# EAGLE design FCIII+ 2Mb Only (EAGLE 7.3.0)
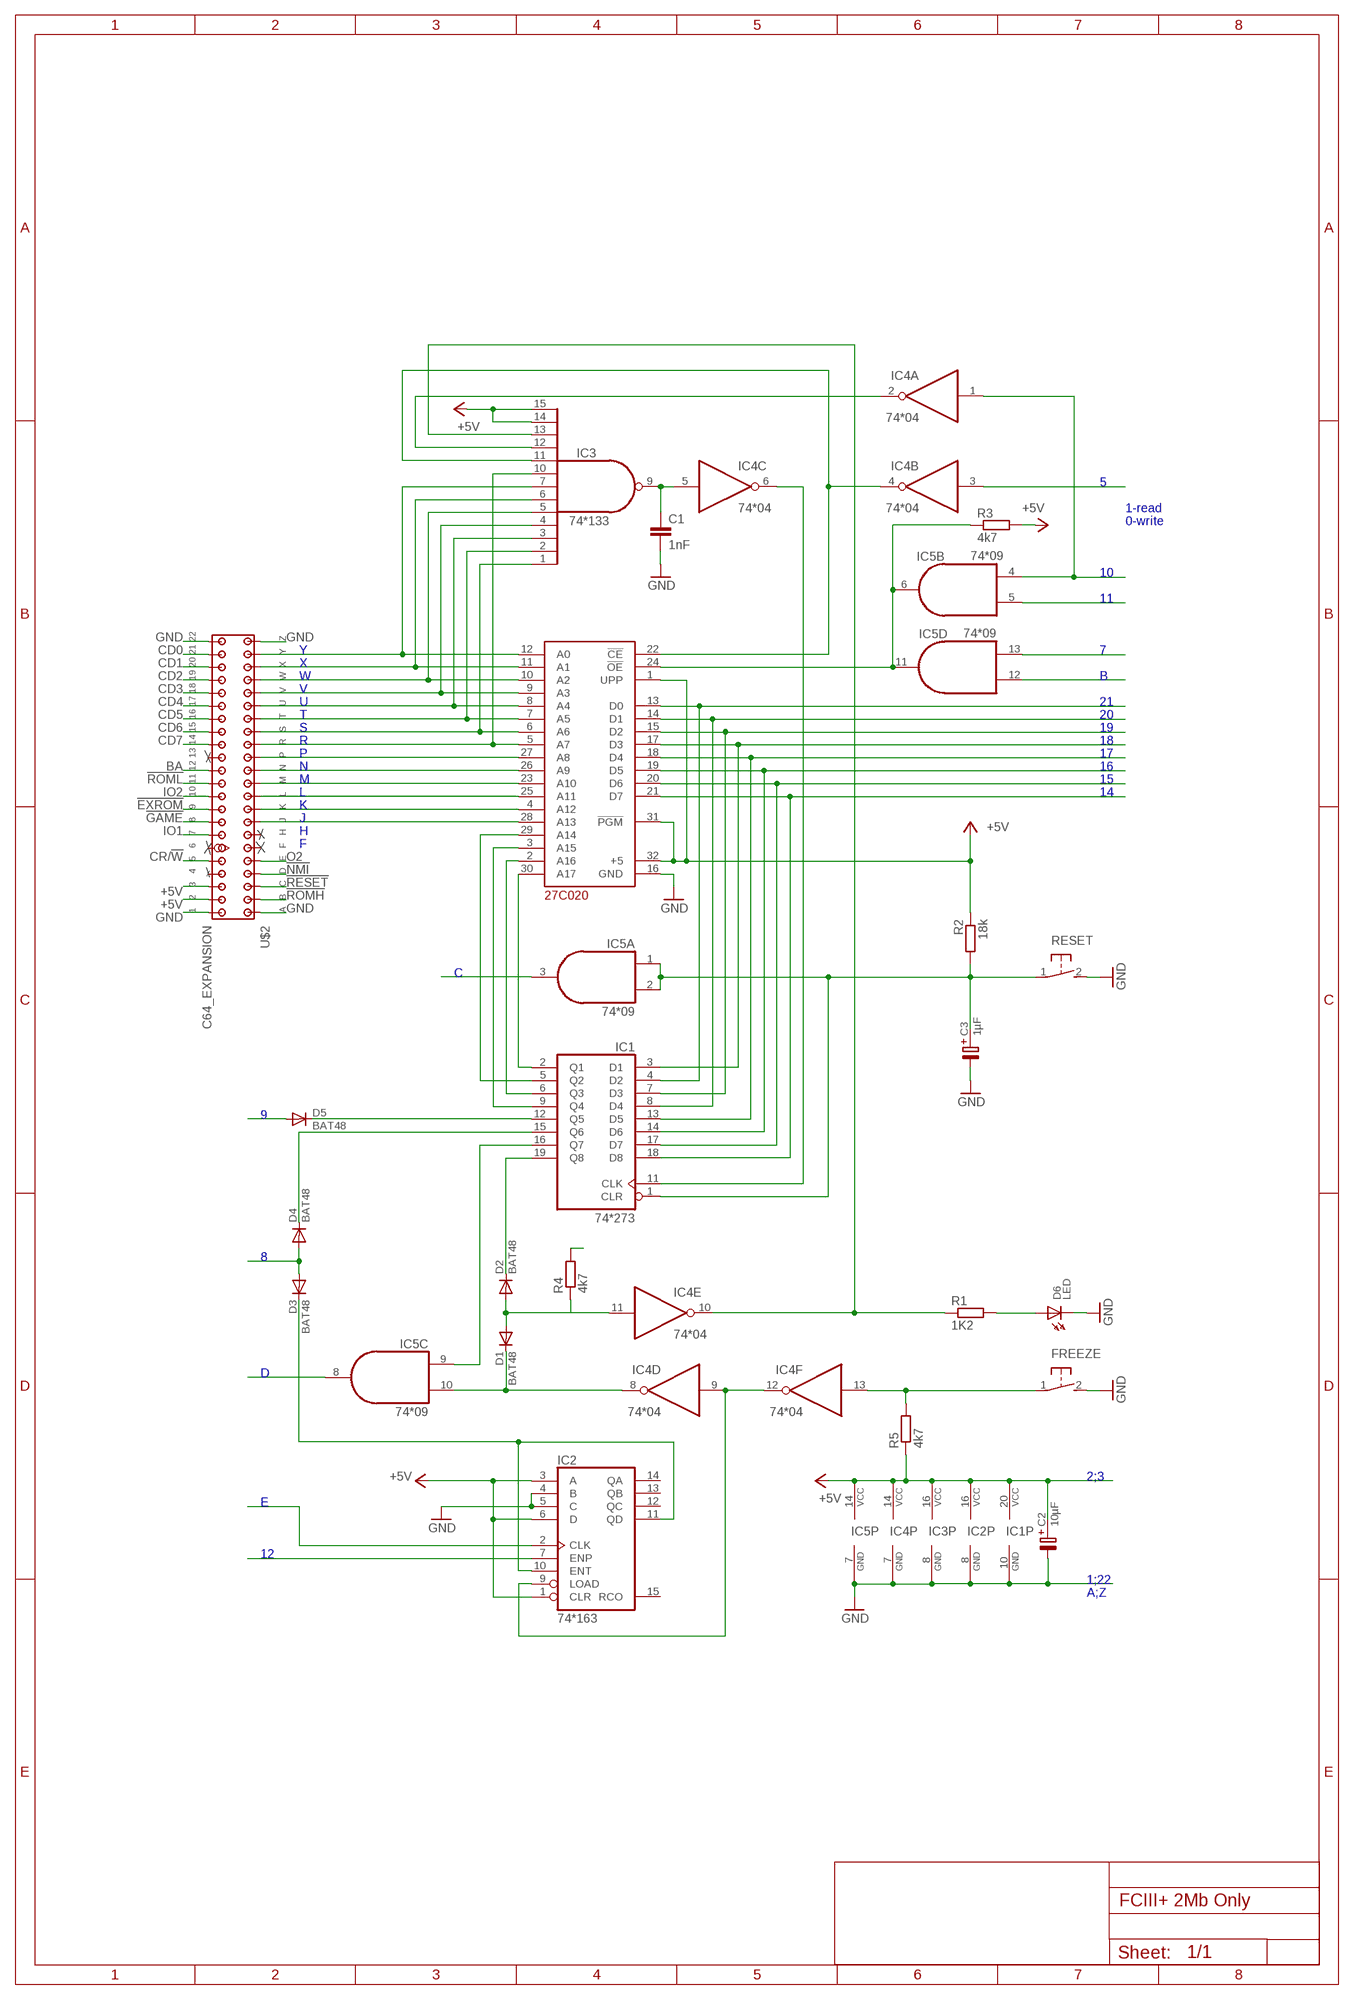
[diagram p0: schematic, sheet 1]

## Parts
C1  1nF  C-EU050-024X044  [C050-024X044]
C2  10µF  E1,6-4  [E1,6-4]
C3  1µF  E1,6-4  [E1,6-4]
D1  BAT48  OA91  [DO07]
D2  BAT48  OA91  [DO07]
D3  BAT48  OA91  [DO07]
D4  BAT48  OA91  [DO07]
D5  BAT48  OA91  [DO07]
D6  LED  LED3E  [LED3E]
FREEZE  31-XX  [B3F-31XX]
IC1  74*273  74273  [DIL20]
IC2  74*163  74160  [DIL16]
IC3  74*133  74133  [DIL16]
IC4  74*04  7404  [DIL14]
IC5  74*09  7409  [DIL14]
R1  1K2  R-EU_0207/10  [0207/10]
R2  18k  R-EU_0207/10  [0207/10]
R3  4k7  R-EU_0207/10  [0207/10]
R4  4k7  R-EU_0207/10  [0207/10]
R5  4k7  R-EU_0207/10  [0207/10]
RESET  31-XX  [B3F-31XX]
U$1  27C020  [DIL32]
U$2  C64_EXPANSION  [EDGE44_254]

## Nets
!EXROM: D5.A U$2.P$9(!EXROM)
!GAME: D3.A D4.A U$2.P$8(!GAME)
!NMI: IC5.8(C:O) U$2.D(!NMI)
!RESET: IC5.3(A:O) U$2.C(!RESET)
!ROMH: IC5.12(D:I0) U$2.B(!ROMH)
!ROML: IC5.5(B:I1) U$2.P$11(!ROML)
+5V: C2.+ IC1.20(VCC) IC2.1(CLR) IC2.3(A) IC2.6(D) IC2.16(VCC) IC3.14(I11) IC3.15(I12) IC3.16(VCC) IC4.14(P:VCC) IC5.14(P:VCC) R2.1 R3.2 R5.1 U$1.1(UPP) U$1.31(!PGM) U$1.32(+5) U$2.P$2(+5V_2) U$2.P$3(+5V_3)
BA: IC2.7(ENP) U$2.P$12(BA)
CA0: IC3.7(I6) U$1.12(A0) U$2.Y(A0)
CA1: IC3.6(I5) U$1.11(A1) U$2.X(A1)
CA2: IC3.5(I4) U$1.10(A2) U$2.W(A2)
CA3: IC3.4(I3) U$1.9(A3) U$2.V(A3)
CA4: IC3.3(I2) U$1.8(A4) U$2.U(A4)
CA5: IC3.2(I1) U$1.7(A5) U$2.T(A5)
CA6: IC3.1(I0) U$1.6(A6) U$2.S(A6)
CA7: IC3.10(I7) U$1.5(A7) U$2.R(A7)
CA8: U$1.27(A8) U$2.P(A8)
CA9: U$1.26(A9) U$2.N(A9)
CA10: U$1.23(A10) U$2.M(A10)
CA11: U$1.25(A11) U$2.L(A11)
CA12: U$1.4(A12) U$2.K(A12)
CA13: U$1.28(A13) U$2.J(A13)
CD0: IC1.4(D2) U$1.13(D0) U$2.P$21(D0)
CD1: IC1.8(D4) U$1.14(D1) U$2.P$20(D1)
CD2: IC1.7(D3) U$1.15(D2) U$2.P$19(D2)
CD3: IC1.3(D1) U$1.17(D3) U$2.P$18(D3)
CD4: IC1.13(D5) U$1.18(D4) U$2.P$17(D4)
CD5: IC1.14(D6) U$1.19(D5) U$2.P$16(D5)
CD6: IC1.17(D7) U$1.20(D6) U$2.P$15(D6)
CD7: IC1.18(D8) U$1.21(D7) U$2.P$14(D7)
CR/!W: IC4.3(B:I) U$2.P$5(R!W)
FREEZE: FREEZE.1(P) IC4.13(F:I) R5.2
GND: C1.2 C2.- C3.- D6.K FREEZE.2(S) IC1.10(GND) IC2.4(B) IC2.5(C) IC2.8(GND) IC3.8(GND) IC4.7(P:GND) IC5.7(P:GND) RESET.2(S) U$1.16(GND) U$2.A(GND_A) U$2.P$1(GND_1) U$2.P$22(GND_22) U$2.Z(GND_Z)
IO1: IC5.13(D:I1) U$2.P$7(!IO1)
IO2: IC4.1(A:I) IC5.4(B:I0) U$2.P$10(!IO2)
N$1: IC1.2(Q1) U$1.30(A17)
N$2: IC2.9(LOAD) IC4.9(D:I) IC4.12(F:O)
N$3: D1.K IC4.8(D:O) IC5.10(C:I1)
N$4: IC1.16(Q7) IC5.9(C:I0)
N$5: D3.K IC2.10(ENT) IC2.11(QD)
N$6: D5.K IC1.12(Q5)
N$7: R4.2
N$9: D1.A D2.A IC4.11(E:I) R4.1
N$10: D2.K IC1.19(Q8)
N$12: D4.K IC1.15(Q6)
N$14: IC1.6(Q3) U$1.2(A16)
N$15: IC1.9(Q4) U$1.3(A15)
N$16: IC1.5(Q2) U$1.29(A14)
N$34: C1.1 IC3.9(O) IC4.5(C:I)
N$35: IC1.11(CLK) IC4.6(C:O)
N$36: IC3.11(I8) IC4.4(B:O) U$1.22(!CE)
N$38: IC3.12(I9) IC4.2(A:O)
N$46: IC5.6(B:O) IC5.11(D:O) R3.1 U$1.24(!OE)
N$47: IC3.13(I10) IC4.10(E:O) R1.1
N$49: D6.A R1.2
O2: IC2.2(CLK) U$2.E(PHI2)
RESET: C3.+ IC1.1(CLR) IC5.1(A:I0) IC5.2(A:I1) R2.2 RESET.1(P)
Unconnected: IC2.12(QC) IC2.13(QB) IC2.14(QA) IC2.15(RCO) U$2.F(A15) U$2.H(A14) U$2.P$4(!IRQ) U$2.P$6(DOTCLK) U$2.P$13(!DMA)

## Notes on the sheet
- 5
- 1-read
- 0-write
- 10
- 11
- Y | 7
- X
- W | B
- V
- U | 21
- T | 20
- S | 19
- R | 18
- P | 17
- N | 16
- M | 15
- L | 14
- K
- J
- H
- F
- C
- 9
- 8
- D
- 2;3
- E
- 12
- 1;22
- A;Z

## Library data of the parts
C1 = rcl:C-EU: CAPACITOR, European symbol
C2 C3 = polcap:E1,6-4
D1-D5 = diode:OA91
D6 = led:LED3E
FREEZE RESET = switch-omron:31-XX: OMRON SWITCH; MPN: B3F-3100; OC_FARNELL: 959704; OC_NEWARK: 36M3582
IC1 = 74xx:74273
IC2 = 74xx:74160
IC3 = 74xx:74133
IC4 = 74xx:7404
IC5 = 74xx:7409
R1-R5 = rcl:R-EU_: RESISTOR, European symbol
U$1 = memory:27C020
U$2 = 000_e5frog:C64_EXPANSION

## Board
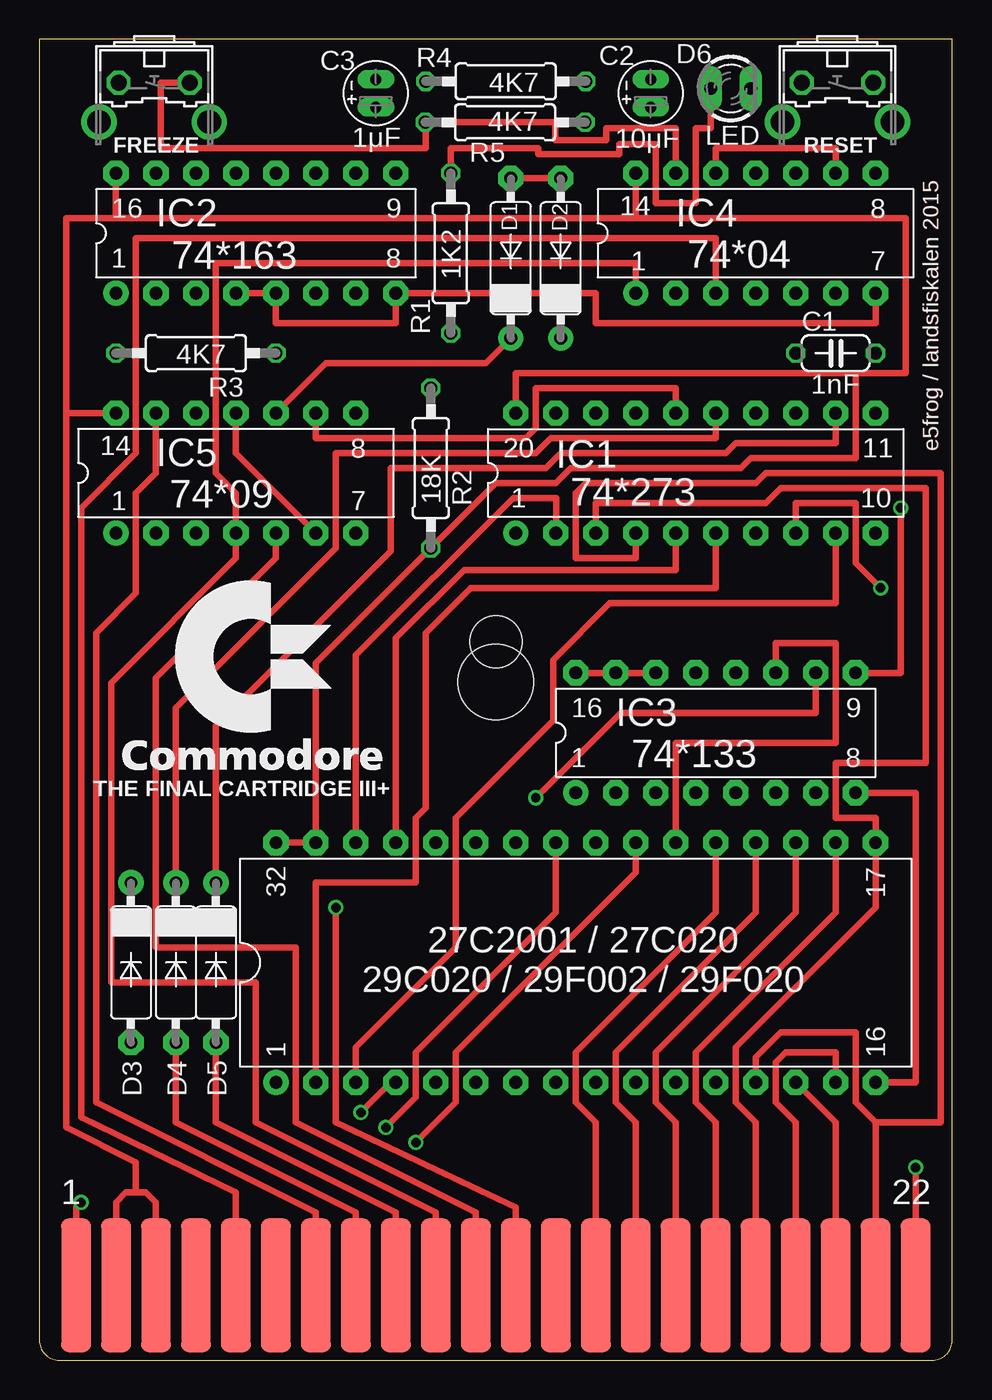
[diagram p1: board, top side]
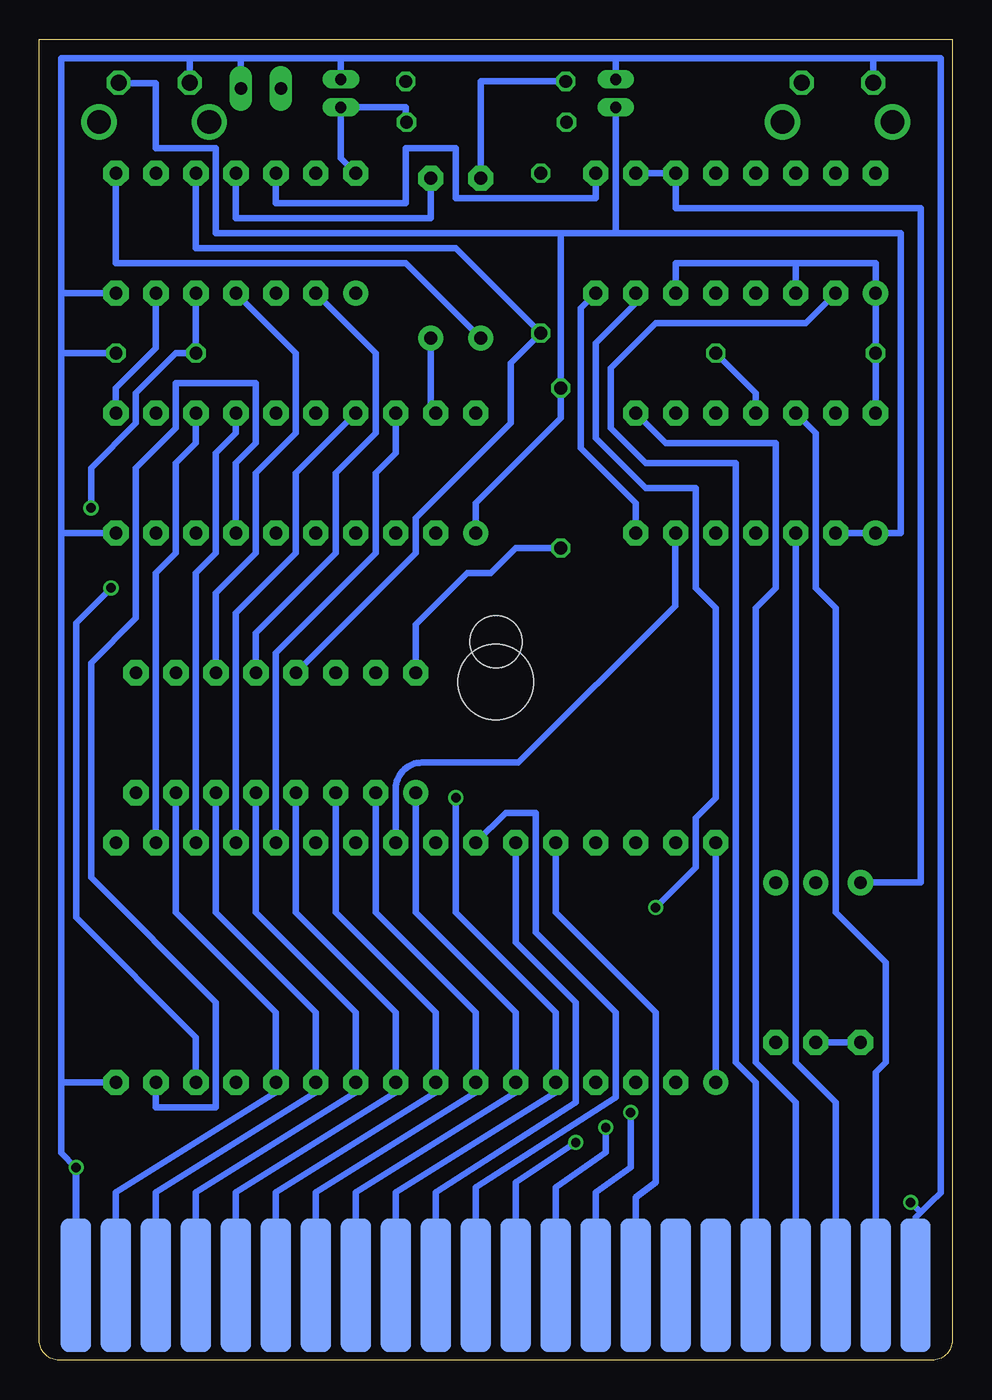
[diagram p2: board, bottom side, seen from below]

Size 58 x 83.95 mm. Coordinates in mm from the lower left corner, seen from the top.
Outline: 0,83.95 0,1.27 arc90 1.27,0 56.73,0 arc90 58,1.27 58,83.95 0,83.95
Copper layers (1*16): Top 0.0356mm / dielectric 1.5011mm / Bottom 0.0356mm
Design rules "oshpark": minimum track width 6mil, minimum drill 13mil, track to track 6mil, track to pad 6mil, pad to pad 6mil, via to via 6mil, smd to smd 6mil, copper to edge 15mil, drill to drill 6mil, minimum pad ring 7mil, minimum via ring 7mil, stop-mask expansion 3mil, vias tented up to drill 0mil, thermal gap 10mil
Holes 4.8 mm at 29,43.1
Holes 3.3 mm at 29,45.65
tRestrict: area 26.2,40.4 to 31.8,45.9; area 26,42.7 to 32,48.7
bRestrict: area 26,40.1 to 32,46.1

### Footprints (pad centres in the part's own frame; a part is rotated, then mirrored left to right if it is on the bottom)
C050-024X044 = drill 0.813 octagon: 1 -2.54,0; 2 2.54,0
E1,6-4 = drill 0.711 pad 1.168 long: + -0.889,0; - 0.889,0
DO07 = drill 0.813 pad 1.6 octagon: A 5.08,0 | drill 0.813 pad 1.6: K -5.08,0
LED3E = drill 0.813 pad 1.422 long: A -1.27,0; K 1.27,0
B3F-31XX = drill 1.016 octagon: 1 -2.261,-1.245; 2 2.261,-1.245 | drill 1.499 pad 2.159: 3 -3.505,1.245; 4 3.505,1.245
DIL20 = drill 0.813 pad 1.6: 1 -11.43,-3.81 | drill 0.813 pad 1.6 octagon: 2 -8.89,-3.81; 3 -6.35,-3.81; 4 -3.81,-3.81; 5 -1.27,-3.81; 6 1.27,-3.81; 7 3.81,-3.81; 8 6.35,-3.81; 9 8.89,-3.81; 10 11.43,-3.81; 11 11.43,3.81; 12 8.89,3.81; 13 6.35,3.81; 14 3.81,3.81; 15 1.27,3.81; 16 -1.27,3.81; 17 -3.81,3.81; 18 -6.35,3.81; 19 -8.89,3.81; 20 -11.43,3.81
DIL16 = drill 0.813 pad 1.6: 1 -8.89,-3.81 | drill 0.813 pad 1.6 octagon: 2 -6.35,-3.81; 3 -3.81,-3.81; 4 -1.27,-3.81; 5 1.27,-3.81; 6 3.81,-3.81; 7 6.35,-3.81; 8 8.89,-3.81; 9 8.89,3.81; 10 6.35,3.81; 11 3.81,3.81; 12 1.27,3.81; 13 -1.27,3.81; 14 -3.81,3.81; 15 -6.35,3.81; 16 -8.89,3.81
DIL14 = drill 0.813 pad 1.6: 1 -7.62,-3.81 | drill 0.813 pad 1.6 octagon: 2 -5.08,-3.81; 3 -2.54,-3.81; 4 0,-3.81; 5 2.54,-3.81; 6 5.08,-3.81; 7 7.62,-3.81; 8 7.62,3.81; 9 5.08,3.81; 10 2.54,3.81; 11 0,3.81; 12 -2.54,3.81; 13 -5.08,3.81; 14 -7.62,3.81
0207/10 = drill 0.813 octagon: 1 -5.08,0; 2 5.08,0
DIL32 = drill 0.813 pad 1.6: 1 -19.05,-7.62 | drill 0.813 pad 1.6 octagon: 2 -16.51,-7.62; 3 -13.97,-7.62; 4 -11.43,-7.62; 5 -8.89,-7.62; 6 -6.35,-7.62; 7 -3.81,-7.62; 8 -1.27,-7.62; 9 1.27,-7.62; 10 3.81,-7.62; 11 6.35,-7.62; 12 8.89,-7.62; 13 11.43,-7.62; 14 13.97,-7.62; 15 16.51,-7.62; 16 19.05,-7.62; 17 19.05,7.62; 18 16.51,7.62; 19 13.97,7.62; 20 11.43,7.62; 21 8.89,7.62; 22 6.35,7.62; 23 3.81,7.62; 24 1.27,7.62; 25 -1.27,7.62; 26 -3.81,7.62; 27 -6.35,7.62; 28 -8.89,7.62; 29 -11.43,7.62; 30 -13.97,7.62; 31 -16.51,7.62; 32 -19.05,7.62
EDGE44_254 = smd 1.9 x 8.5 bottom: A 54.29,-4.25; B 51.75,-4.25; C 49.21,-4.25; D 46.67,-4.25; E 44.13,-4.25; F 41.59,-4.25; H 39.05,-4.25; J 36.51,-4.25; K 33.97,-4.25; L 31.43,-4.25; M 28.89,-4.25; N 26.35,-4.25; P 23.81,-4.25; R 21.27,-4.25; S 18.73,-4.25; T 16.19,-4.25; U 13.65,-4.25; V 11.11,-4.25; W 8.57,-4.25; X 6.03,-4.25; Y 3.49,-4.25; Z 0.95,-4.25 | smd 1.9 x 8.5: P$1 54.29,-4.25; P$2 51.75,-4.25; P$3 49.21,-4.25; P$4 46.67,-4.25; P$5 44.13,-4.25; P$6 41.59,-4.25; P$7 39.05,-4.25; P$8 36.51,-4.25; P$9 33.97,-4.25; P$10 31.43,-4.25; P$11 28.89,-4.25; P$12 26.35,-4.25; P$13 23.81,-4.25; P$14 21.27,-4.25; P$15 18.73,-4.25; P$16 16.19,-4.25; P$17 13.65,-4.25; P$18 11.11,-4.25; P$19 8.57,-4.25; P$20 6.03,-4.25; P$21 3.49,-4.25; P$22 0.95,-4.25

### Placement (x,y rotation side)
C1  50.59,64 0 top
C2  38.84,80.52 90 top
C3  21.38,80.52 90 top
D1  29.95,70.04 90 top
D2  33.13,70.04 90 top
D3  5.82,25.27 270 top
D4  8.68,25.27 270 top
D5  11.22,25.27 270 top
D6  43.92,80.83 0 top
FREEZE  7.29,79.95 180 top
IC1  41.7,56.38 0 top
IC2  13.76,71.62 0 top
IC3  42.97,39.88 0 top
IC4  45.51,71.62 0 top
IC5  12.49,56.38 0 top
R1  26.14,70.36 90 top
R2  24.87,56.7 90 top
R3  9.95,64 180 top
R4  29.64,81.28 0 top
R5  29.59,78.68 180 top
RESET  50.71,79.95 180 top
U$1  34.08,25.27 0 top
U$2  56.62,0.51 180 top

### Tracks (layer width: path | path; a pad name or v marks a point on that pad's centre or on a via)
!EXROM
  Top 0.406: D5.A 11.22,15.11 22.65,9.39 U$2.P$9
!GAME
  Top 0.406: D4.A 8.68,15.11 20.11,9.39 U$2.P$8
  Bottom 0.406: D3.A D4.A
!NMI
  Bottom 0.406: IC5.8 18.2,58.29 11.22,58.29 11.22,49.08 12.49,47.81 12.49,18.92 9.95,16.38 U$2.D
!RESET
  Bottom 0.406: IC5.3 9.95,18.92 7.41,16.38 U$2.C
!ROMH
  Bottom 0.406: IC5.12 8.68,58.92 8.68,49.08 7.41,47.81 7.41,28.45 4.24,25.27 4.24,18.92 4.87,18.29 U$2.B
!ROML
  Top 0.406: U$2.P$11 27.73,9.39 16.3,15.11 16.3,26.22 7.41,26.22 7.41,32.89 7.41,43.37 15.03,50.99 IC5.5
+5V
  Top 0.406: IC1.20 30.27,62.73 51.86,62.73 | 51.86,62.73 55.03,62.73 55.03,72.58 37.89,72.58 | 37.89,72.58 IC4.14 | 4.87,72.58 IC2.16 | 4.87,72.58 37.89,72.58 | 4.87,72.58 1.7,72.58 1.7,60.2 | 1.7,60.2 IC5.14 | 1.7,60.2 1.7,14.79 6.14,12.57 6.14,10.66 | U$2.P$2 4.87,10.03 5.5,10.66 6.14,10.66 | 6.14,10.66 6.78,10.66 7.41,10.03 U$2.P$3 | IC3.16 IC3.15 IC3.14 | 51.86,62.73 51.86,57.34 45.19,57.34 44.56,56.7 33.76,56.7 32.81,55.75 29,55.75 R2.1 17.57,44.32 U$1.31 U$1.32
  Bottom 0.406: U$1.32 U$1.1 | 9.95,69.72 4.87,69.72 IC2.1 R3.2 IC5.14 | 9.95,69.72 IC2.3 | IC3.16 34.08,46.76 30.8,50.04 29.31,50.04 27.73,51.62 R2.1 | IC4.14 38.84,76.39 C2.+ | IC2.6 17.57,69.72 9.95,69.72 | 38.84,79.5 C2.+ | R5.1 34.72,78.68 34.72,79.63 C2.+
BA  (via drill 0.6)
  Top 0.406: U$2.P$12 30.27,9.71 18.84,15.11 18.84,15.43 v18.84,28.76
  Bottom 0.406: IC2.7 20.11,67.18 22.65,64.64 22.65,58.61 19.48,55.43 16.3,55.43 16.3,49.08 15.03,47.81 15.03,35.75 16.3,34.48 16.3,31.3 v18.84,28.76
CA0
  Bottom 0.406: U$2.Y 53.13,10.66 42.97,17.02 U$1.12 42.97,22.09 49.32,28.45 IC3.7
CA1
  Bottom 0.406: U$2.X 50.59,10.66 40.43,17.02 U$1.11 40.43,22.09 46.78,28.45 IC3.6
CA2
  Bottom 0.406: U$2.W 48.05,10.66 37.89,17.02 U$1.10 37.89,22.09 44.24,28.45 IC3.5
CA3
  Bottom 0.406: U$2.V 45.51,10.66 35.35,17.02 U$1.9 35.35,22.09 41.7,28.45 IC3.4
CA4
  Bottom 0.406: U$2.U 42.97,10.66 32.81,17.02 U$1.8 32.81,22.09 39.16,28.45 IC3.3
CA5
  Bottom 0.406: U$2.T 40.43,10.66 30.27,17.02 U$1.7 30.27,22.09 36.62,28.45 IC3.2
CA6
  Bottom 0.406: U$2.S 37.89,10.66 27.73,17.02 U$1.6 27.73,22.09 34.08,28.45 IC3.1
CA7  (via drill 0.6)
  Top 0.406: v31.54,35.75 36.94,41.15 49.32,41.15 IC3.10
  Bottom 0.406: U$2.R 35.35,10.66 25.19,17.02 U$1.5 25.19,22.09 26.46,23.36 31.54,28.45 v31.54,35.75
CA8
  Bottom 0.406: U$1.27 27.73,26.54 23.92,22.73 23.92,16.38 32.81,10.66 U$2.P
CA9
  Bottom 0.406: U$1.26 28.36,34.8 26.46,34.8 26.46,27.18 25.19,25.91 21.38,22.09 21.38,16.7 30.27,10.98 U$2.N
CA10  (via drill 0.6)
  Top 0.406: v23.92,13.84 26.46,16.38 26.46,19.55 37.89,30.98 U$1.23
  Bottom 0.406: v23.92,13.84 27.73,11.3 U$2.M
CA11  (via drill 0.6)
  Top 0.406: v22.02,14.79 23.92,16.7 23.92,19.55 32.81,28.45 U$1.25
  Bottom 0.406: v22.02,14.79 22.02,13.21 25.19,10.98 U$2.L
CA12  (via drill 0.6)
  Top 0.406: v20.43,15.74 22.33,17.65 U$1.4
  Bottom 0.406: v20.43,15.74 20.43,12.25 22.65,10.66 U$2.K
CA13
  Bottom 0.406: U$2.J 20.11,10.35 18.84,11.3 18.84,22.09 25.19,28.45 U$1.28
CD0
  Top 0.406: 53.13,15.11 51.86,16.38 51.86,20.82 47.1,20.82 45.51,19.24 U$1.13 | 53.13,15.11 U$2.P$21 | IC1.4 37.89,50.99 34.08,50.99 34.08,55.12 34.72,55.75 45.51,55.75 46.15,56.38 57.26,56.38 57.26,15.11 53.13,15.11
CD1  (via drill 0.6)
  Top 0.406: U$1.14 50.59,15.11 U$2.P$20 | IC1.8 48.05,54.48 51.86,54.48 51.86,50.67 v53.45,49.08
  Bottom 0.406: U$1.14 48.05,20.51 55.67,28.13 55.67,46.86 v53.45,49.08
CD2
  Top 0.406: U$1.15 50.59,19.55 47.41,19.55 46.78,18.92 46.78,16.38 48.05,15.11 U$2.P$19
  Bottom 0.406: U$1.15 50.59,16.06 46.78,16.06 46.78,22.73 54.72,30.67 54.72,44.32 51.86,47.18 51.86,56.7 49.32,59.24 49.32,60.83 49.32,62.1 44.24,62.1 44.24,61.47 44.24,58.29 45.51,57.02 IC1.7
CD3
  Top 0.406: IC1.3 35.35,54.48 46.15,54.48 47.1,55.43 56.3,55.43 56.3,37.97 50.59,37.97 50.59,34.48 53.13,34.48 U$1.17 53.13,28.76 44.24,19.87 44.24,16.38 45.51,15.11 U$2.P$18
CD4
  Top 0.406: U$1.18 50.59,28.45 41.7,19.55 41.7,16.38 42.97,15.11 U$2.P$17
  Bottom 0.406: IC1.13 48.05,58.29 49.32,57.02 49.32,51.3 50.59,50.03 U$1.18
CD5
  Top 0.406: U$1.19 48.05,28.45 39.16,19.55 39.16,16.38 40.43,15.11 U$2.P$16
  Bottom 0.406: IC1.14 45.51,58.92 46.78,57.66 46.78,51.3 48.05,50.03 U$1.19
CD6
  Top 0.406: U$1.20 45.51,31.62 45.51,28.45 36.62,19.55 36.62,16.38 37.89,15.11 U$2.P$15
  Bottom 0.406: U$1.20 45.51,45.27 45.51,47.49 41.7,51.3 41.7,56.38 IC1.17
CD7
  Top 0.406: U$1.21 42.97,31.62 42.97,28.45 34.08,19.55 34.08,16.38 35.35,15.11 U$2.P$14
  Bottom 0.406: U$1.21 42.97,44.95 36.62,51.3 36.62,56.38 35.35,57.66 IC1.18
CR/!W
  Top 0.406: IC4.3 42.97,71.31 6.14,71.31 6.14,57.66 2.65,54.16 2.65,15.43 12.49,10.66 U$2.P$5
FREEZE
  Top 0.406: FREEZE.1 7.73,81.19 7.73,77.02 24.55,77.02 24.55,78.29 24.51,78.29 R5.2 32.77,78.68 32.77,77.53 36.01,77.53 36.01,78.29 40.43,78.29 IC4.13
GND  (via drill 0.6)
  Top 0.406: IC4.7 53.13,65.91 35.35,65.91 35.35,67.81 IC2.8 22.65,65.91 15.03,65.91 IC2.5 IC2.4 | U$2.P$1 2.33,9.71 v2.65,10.03 | U$2.P$22 55.67,10.35 v55.67,12.25 | IC3.8 55.67,36.06 55.67,17.65 U$1.16
  Bottom 0.406: 21.38,82.74 38.84,82.74 | 38.84,82.74 45.19,82.74 | 21.38,82.74 14.47,82.74 8.04,82.74 5.19,82.74 | 45.19,82.74 D6.K | 45.19,82.74 45.75,82.74 48.37,82.74 | 48.37,82.74 50.03,82.74 56.62,82.74 56.62,67.81 | 56.62,64 C1.2 | 56.62,67.81 56.62,64 | 56.62,64 56.62,52.58 | 56.62,17.65 56.62,13.17 55.67,12.22 U$2.P$22 55.67,10.35 v55.67,12.25 | 56.62,52.58 56.62,37.65 56.62,17.65 | 56.62,17.65 U$1.16 | 21.38,82.74 C3.- | IC2.8 23.6,66.86 23.6,57.97 20.11,54.48 IC5.7 | 56.62,67.81 IC4.7 | 5.19,82.74 0.74,82.74 0.74,10.63 1.38,10.03 2.01,9.39 | 56.62,52.58 IC1.10 | 2.01,9.39 2.33,9.08 | 2.33,9.08 U$2.P$1 | U$2.P$1 | v2.65,10.03 2.01,9.39 | 2.01,9.39 2.33,9.08 | 2.33,9.08 U$2.P$1 | C2.- 38.84,82.74 | FREEZE.2 5.03,82.58 5.19,82.74 | RESET.2 48.45,82.66 48.37,82.74
IO1
  Top 0.406: IC5.13 7.41,56.38 6.14,55.12 6.14,48.77 3.6,46.23 3.6,33.84 3.6,16.38 17.57,9.39 U$2.P$7
IO2
  Top 0.406: IC4.1 37.89,69.72 11.22,69.72 11.22,56.38 12.49,55.12 IC5.4 12.49,50.99 4.55,43.05 4.55,32.57 4.55,24 13.76,24 13.76,15.11 25.19,9.39 U$2.P$10
N$1
  Top 0.406: U$1.30 20.11,44.81 30.1,54.8 32.83,54.8 32.83,52.59 IC1.2
N$2
  Top 0.406: IC4.12 42.97,77.02 50.59,77.02 IC4.9
  Bottom 0.406: IC4.12 42.97,73.53 34.72,73.53 34.72,77.02 31.54,77.02 31.54,73.85 27.41,73.85 22.65,73.85 IC2.9
N$3
  Top 0.406: IC5.10 18.2,63.37 28.36,63.37 D1.K
  Bottom 0.406: D1.K 34.72,69.72 47.41,69.72 53.13,69.72 53.13,73.85 IC4.8
N$4
  Top 0.406: IC5.9 17.57,58.61 30.91,58.61 31.54,59.24 31.54,61.78 40.43,61.78 IC1.16
N$5
  Bottom 0.406: IC2.10 IC2.11 17.57,73.21 2.01,73.21 2.01,30.35 D3.K
N$6
  Top 0.406: D5.K 11.22,31.94 11.22,40.32 22.33,51.43 22.33,56.7 32.17,56.7 33.13,57.66 43.6,57.66 44.24,58.29 50.59,58.29 IC1.12
N$9
  Top 0.406: D1.A D2.A
  Bottom 0.406: D2.A 33.13,72.58 45.51,72.58 IC4.11 | D1.A 29.95,81.28 R4.1
N$10
  Bottom 0.406: IC1.19 33.13,60.83 D2.K
N$12
  Top 0.406: IC1.15 42.97,58.61 32.49,58.61 31.54,57.66 18.84,57.66 18.84,51.62 8.68,41.46 8.68,32.57 D4.K
N$14
  Top 0.406: IC1.6 42.97,49.08 27.41,49.08 24.55,46.23 24.55,35.11 23.92,34.48 23.92,30.35 22.02,30.35 17.57,30.35 U$1.2
N$15
  Top 0.406: IC1.9 50.59,48.13 36.26,48.13 32.64,44.51 32.64,40.66 26.46,34.48 26.46,26.22 20.11,19.87 U$1.3
N$16
  Top 0.406: U$1.29 22.65,45.89 26.99,50.23 40.45,50.23 40.45,52.56 IC1.5
N$34  (via drill 0.6)
  Top 0.406: IC3.9 54.72,43.69 v54.72,54.16
  Bottom 0.406: IC4.5 C1.1 49.32,64 51.86,61.47 51.86,59.56 54.72,56.7 v54.72,54.16
N$35
  Bottom 0.406: IC1.11 53.13,61.78 50.59,64.32 IC4.6
N$36
  Top 0.406: U$1.22 40.43,34.48 40.43,39.24 48.05,39.24 50.59,39.24 50.59,45.59 46.78,45.59 IC3.11
  Bottom 0.406: IC4.4 41.7,64 41.7,59.56 41.7,59.24 41.7,58.92 44.24,56.38 44.24,51.94 44.24,51.3 46.78,48.77 IC3.11
N$38
  Bottom 0.406: IC4.2 36.62,64 36.62,58.92 39.16,56.38 39.16,51.3 44.24,46.23 IC3.12
N$46
  Top 0.406: IC5.11 12.49,57.66 IC5.6
  Bottom 0.406: IC5.11 12.49,61.47 R3.1 | U$1.24 35.35,36.34 arc90 33.72,37.97 27.56,37.97 17.59,47.94 17.59,52.56 IC5.6
N$47
  Bottom 0.406: IC3.13 40.11,45.27 34.08,51.3 34.08,53.53 28.05,59.56 28.05,63.37 R1.1 31.54,70.67 48.05,70.67 48.05,73.85 IC4.10
N$49
  Top 0.406: R1.2 26.14,77.02 31.69,77.02 31.69,76.64 36.83,76.64 36.83,77.28 39.16,77.28 39.16,73.53 41.7,73.53 41.7,78.29 42.65,78.29 D6.A
O2
  Bottom 0.406: IC2.2 9.31,65.91 18.84,65.91 21.7,63.05 21.7,59.24 19.48,57.02 13.76,57.02 13.76,18.92 12.49,17.65 U$2.E
RESET
  Bottom 0.406: C3.+ 21.38,79.21 21.38,77.3 21.38,71.62 | 21.38,71.62 24.87,71.62 | 24.87,71.62 R2.2 24.87,59.88 30.27,54.48 IC1.1 | IC5.1 IC5.2 3.28,52.58 3.28,71.62 21.38,71.62 | 24.87,71.62 46.78,71.62 46.78,74.48 46.78,77.02 50.59,77.02 50.59,81.15 52.97,81.15 RESET.1

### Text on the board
Top: e5frog / landsfiskalen 2015
tNames: 4K7 | 4K7 | LED | 1μF | 10μF | 74*163 | 1K2 | 74*04 | 4K7 | 1nF | e5frog / landsfiskalen 2015 | 74*09 | 18K | 74*273 | 74*133 | THE FINAL CARTRIDGE III+ | 27C2001 / 27C020 / 29C020 / 29F002 / 29F020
